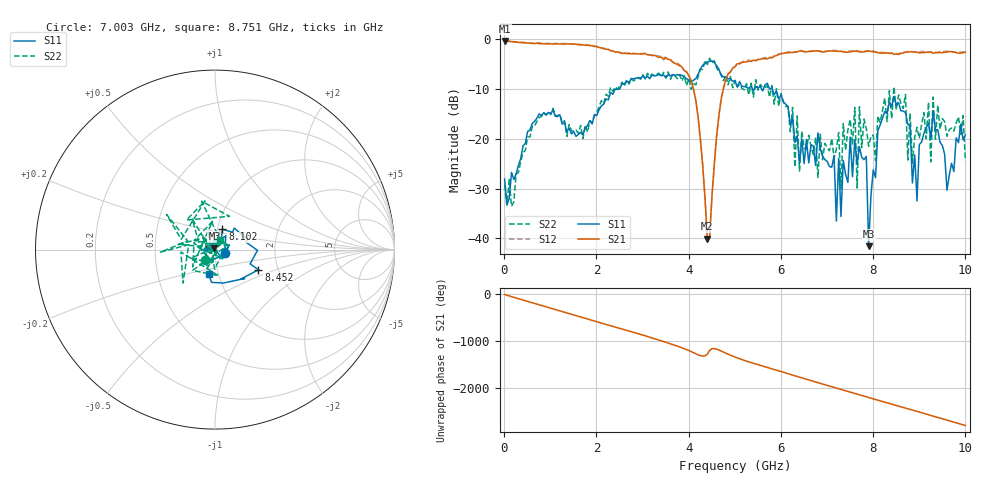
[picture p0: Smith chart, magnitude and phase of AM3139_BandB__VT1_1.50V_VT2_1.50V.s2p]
! Date/Time: Tue, Nov 13, 2018 4:59 PM
! Network Analyzer: Agilent Technologies E8364B Rev: A.07.50.67
! Sweep from 0.010 to 10.000 GHz, 201 Points, Sweep Type: LIN
! Power Supply: 1.500 V, 0.000 A
# Hz S DB R 50
!freq MagS11 AngS11 MagS21 AngS21 MagS12 AngS12 MagS22 AngS22
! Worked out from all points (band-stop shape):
!   201 points, 10 MHz to 10 GHz, reference 50 ohm
!   highest |S21| = -0.30 dB at 10 MHz (marker M1); lowest = -40.1 dB at 4.406 GHz (marker M2)
!   |S21| within 3 dB of the highest: start of sweep to 3.287 GHz; 5.881 GHz to end of sweep
!   lowest |S11| = -41.6 dB at 7.902 GHz (marker M3), VSWR 1.02, Z = 49.7 + j0.755 ohm
!   |S11| at or under -10 dB: start of sweep to 2.407 GHz; 2.42 GHz to 2.484 GHz (63.92 MHz wide, 2.61 % of centre); 5.813 GHz to end of sweep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
!   |S22| runs from -33.6 to -3.8 dB; largest |S21 - S12| = 0.035
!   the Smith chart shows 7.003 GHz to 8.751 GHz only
!   S11 on the Smith chart (normalised r, x): 7.003 GHz: 1.12, -0.05; 8.102 GHz: 1.06, +0.24; 8.452 GHz: 1.58, -0.38; 8.751 GHz: 0.90, -0.25
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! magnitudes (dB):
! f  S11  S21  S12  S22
! 10 MHz  -28.1  -0.3  -0.2  -29.3
! 1.708 GHz  -19.2  -1.1  -1.0  -19.9
! 3.357 GHz  -7.0  -3.6  -3.4  -6.8
! 4.106 GHz  -8.2  -9.9  -10.1  -8.9
! 4.406 GHz  -4.5  -40.1  -39.9  -5.1
! 5.005 GHz  -8.3  -5.4  -5.5  -8.2
! 6.703 GHz  -21.4  -2.4  -2.2  -23.1
! 7.003 GHz  -24.5  -2.4  -2.4  -21.8
! 7.203 GHz  -36.6  -2.4  -2.2  -22.0
! 7.253 GHz  -23.9  -2.4  -2.3  -18.7
! 7.303 GHz  -35.6  -2.4  -2.4  -30.1
! 7.852 GHz  -23.5  -2.4  -2.3  -18.0
! 7.902 GHz  -41.6  -2.3  -2.3  -21.5
! 8.102 GHz  -18.4  -2.7  -2.6  -15.4
! 8.352 GHz  -12.5  -2.8  -2.8  -10.3
! 8.452 GHz  -11.5  -3.0  -2.9  -9.5
! 8.751 GHz  -17.0  -2.5  -2.4  -24.3
! 8.951 GHz  -32.5  -2.6  -2.5  -17.7
! 9.251 GHz  -20.0  -2.5  -2.5  -24.6
! 9.301 GHz  -14.3  -2.8  -2.6  -11.6
! 9.6 GHz  -30.4  -2.5  -2.4  -19.5
! 10 GHz  -19.2  -2.5  -2.4  -24.4
